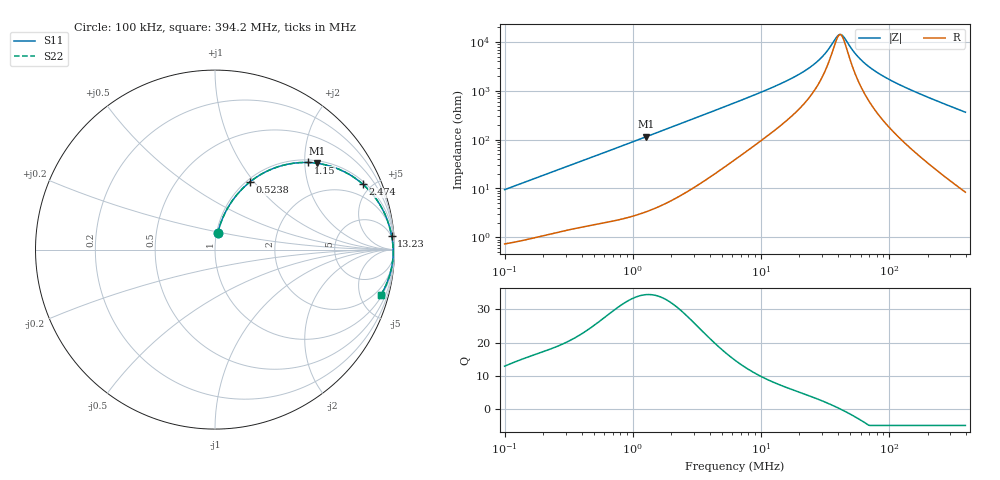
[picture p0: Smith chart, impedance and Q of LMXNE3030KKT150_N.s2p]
! LMXNE3030KKT150_N  S-PARAMETER MODEL  ( General Type )
! Model Generated by TAIYO YUDEN Corporation (https://www.yuden.co.jp/en/)
! Version 1.0
! TAIYO YUDEN Control No. 191023NI43SB-FBB
! Copyright(c) 2019 TAIYO YUDEN CO.,LTD. All Rights Reserved.
! Product Description (link to TY-COMPAS)
! https://ds.yuden.co.jp/TYCOMPAS/or/detail?pn=LMXNE3030KKT150MN&u=M
! Products Name : Inductors
! Characteristics :
!  Inductance : 15 uH , SRF(min) : 25 MHz , DC Resistance(max) : 0.66 Ohm
!  Rated Current : Saturation :450 mA , Temp Rise : 480 mA (40 degC)
!  Case Size : 3.0 x 3.0 / 0.118 x 0.118 [mm/inch] , Thickness : 1 / 0.039 [mm/inch]
!  (Conditions: Temperature = 25 degC , DC Bias Current/Voltage = 0A / 0V)
! External Node Assignments :
!  1  o---GGG---o  2
! GND o---------o GND
! Frequency Range : 0.1MHz  -  394.189695MHz  [ 402 STEP ]
# MHz S RI R 50
! Freq[MHz].  S11 Real  S11 Imag  S21 Real  S21 Imag  S12 Real  S12 Imag  S22 Real  S22 Imag
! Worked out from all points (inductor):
!   401 points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, 100 kHz to 394.2 MHz, reference 50 ohm
!   read as one part in series: L = 14.9 uH near 104.2 kHz
!   highest Q = 34.4 at 1.275 MHz (marker M1), where L = 14.3 uH
!   self-resonance near 41.29 MHz
!   S11 on the Smith chart (normalised r, x): 100 kHz: 1.01, +0.19; 523.8 kHz: 1.04, +0.95; 1.15 MHz: 1.06, +2.07; 2.474 MHz: 1.15, +4.45; 13.23 MHz: 4, +25; 394.2 MHz: 1.17, -7.29
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0.1  0.0159 0.092  0.9841 -0.092  0.9841 -0.092  0.0159 0.092
0.224172  0.0514 0.1948  0.9486 -0.1948  0.9486 -0.1948  0.0514 0.1948
0.400203  0.1285 0.3133  0.8715 -0.3133  0.8715 -0.3133  0.1285 0.3133
0.523771  0.1939 0.3764  0.8061 -0.3764  0.8061 -0.3764  0.1939 0.3764
0.808939  0.3527 0.4621  0.6473 -0.4621  0.6473 -0.4621  0.3527 0.4621
1.150093  0.5175 0.4853  0.4825 -0.4853  0.4825 -0.4853  0.5175 0.4853
1.275497  0.5672 0.4812  0.4328 -0.4812  0.4328 -0.4812  0.5672 0.4812
1.601627  0.6707 0.4555  0.3293 -0.4555  0.3293 -0.4555  0.6707 0.4555
2.473636  0.8241 0.364  0.1759 -0.364  0.1759 -0.364  0.8241 0.364
3.742149  0.9095 0.2654  0.0905 -0.2654  0.0905 -0.2654  0.9095 0.2654
6.278453  0.9597 0.1655  0.0403 -0.1655  0.0403 -0.1655  0.9597 0.1655
13.22715  0.9841 0.0756  0.0159 -0.0756  0.0159 -0.0756  0.9841 0.0756
19.19874  0.9889 0.0465  0.0111 -0.0465  0.0111 -0.0465  0.9889 0.0465
25.12657  0.991 0.029  0.009 -0.029  0.009 -0.029  0.991 0.029
31.55115  0.9922 0.0155  0.00778 -0.0155  0.00778 -0.0155  0.9922 0.0155
39.61841  0.9929 0.00257  0.00705 -0.00257  0.00705 -0.00257  0.9929 0.00257
42.15653  0.9931 -0.000946  0.00693 0.000946  0.00693 0.000946  0.9931 -0.000946
62.46847  0.993 -0.0241  0.00698 0.0241  0.00698 0.0241  0.993 -0.0241
76.83401  0.9923 -0.0376  0.00765 0.0376  0.00765 0.0376  0.9923 -0.0376
100.5574  0.9906 -0.0576  0.00945 0.0576  0.00945 0.0576  0.9906 -0.0576
183.2747  0.9795 -0.119  0.0205 0.119  0.0205 0.119  0.9795 -0.119
394.1897  0.925 -0.2521  0.075 0.2521  0.075 0.2521  0.925 -0.2521
